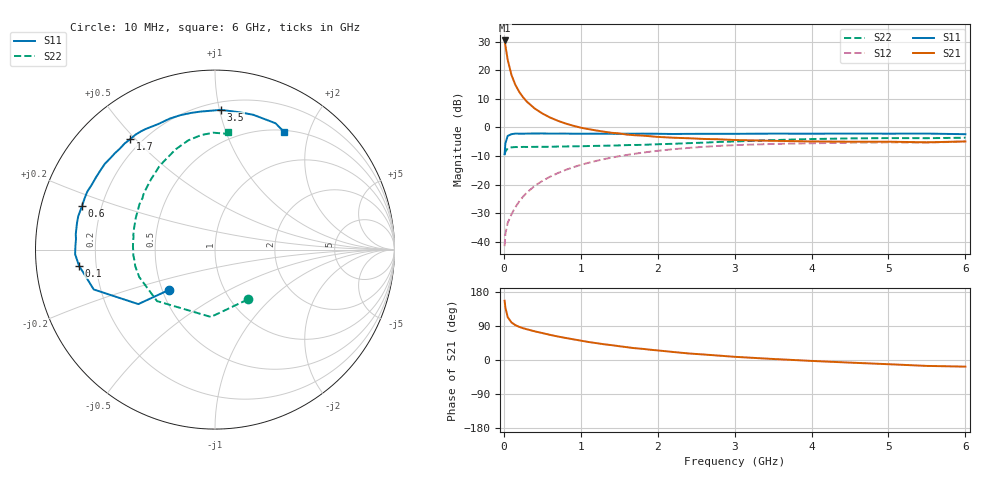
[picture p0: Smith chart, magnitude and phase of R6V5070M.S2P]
! SIEMENS Small Signal Semiconductors
! BFR193
! Si NPN RF Bipolar Junction Transistor in SOT23
! VCE = 0.5 V  IC = 70 mA
! Common Emitter S-Parameters:  May  1996
# GHz  S  MA  R  50
!  f  S11  S21  S12  S22
! GHz  MAG  ANG  MAG  ANG  MAG  ANG  MAG  ANG
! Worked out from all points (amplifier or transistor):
!   36 points, 10 MHz to 6 GHz, reference 50 ohm
!   highest |S21| = 30.4 dB at 10 MHz (marker M1)
!   |S21| within 3 dB of that: start of sweep to 27.83 MHz
!   unconditionally stable (mu >= 1): start of sweep to 18.99 MHz; 95.16 MHz to end of sweep
!   at 250 MHz: K = 1.18, MAG = 14.8 dB, |S12| = -24.2 dB
!   at 1.4 GHz: K = 1.12, MAG = 2.3 dB, |S12| = -10.6 dB
!   at 6 GHz: K = 1.03, MAG = -1.1 dB, |S12| = -4.9 dB
!   S11 on the Smith chart (normalised r, x): 10 MHz: 0.54, -0.28; 100 MHz: 0.13, -0.06; 600 MHz: 0.13, +0.16; 1.7 GHz: 0.16, +0.48; 3.5 GHz: 0.25, +1.01; 6 GHz: 0.52, +1.62
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0.01  0.3393 -138.7  33.13 156.3  0.0084 59.3  0.3324 -56.7
0.02  0.5242 -144.6  27.31 138.5  0.0138 56.2  0.3759 -93.5
0.05  0.7112 -161.8  15.24 113.1  0.0214 51.0  0.432 -138.4
0.1  0.7631 -173.3  8.196 98.9  0.0304 57.4  0.4488 -160.0
0.15  0.7797 -178.1  5.542 92.0  0.0404 63.4  0.4539 -168.2
0.2  0.7778 178.3  4.186 87.4  0.0508 66.5  0.4531 -172.8
0.25  0.7767 175.7  3.361 83.9  0.0617 68.3  0.4565 -176.1
0.3  0.7806 173.6  2.816 81.1  0.0729 69.3  0.4555 -178.6
0.4  0.7832 168.9  2.147 75.7  0.0947 69.5  0.4576 177.7
0.5  0.7843 166.2  1.754 71.1  0.116 69.0  0.4583 174.5
0.6  0.7796 161.9  1.492 66.4  0.1373 67.6  0.4591 171.7
0.7  0.7807 158.4  1.309 62.1  0.1588 66.2  0.4628 169.3
0.8  0.7814 155.5  1.174 58.3  0.1802 64.3  0.465 166.9
1.1  0.7761 145.3  0.934 47.5  0.2408 58.6  0.4726 160.1
1.3  0.7742 138.9  0.843 41.6  0.2788 54.3  0.4785 155.5
1.7  0.7759 127.4  0.731 31.2  0.3458 45.9  0.4937 146.7
2.2  0.7676 114.3  0.661 21.2  0.4162 35.5  0.5174 136.4
2.8  0.7731 100.0  0.62 11.5  0.4761 24.0  0.5578 123.9
3.5  0.7793 87.6  0.583 2.7  0.5146 11.8  0.6002 111.4
4.5  0.7808 74.2  0.563 -6.9  0.5403 -1.2  0.6429 96.9
5.5  0.7805 64.4  0.549 -15.6  0.5435 -12.3  0.6488 83.6
6  0.7612 59.8  0.569 -17.5  0.5664 -15.8  0.6606 83.9
